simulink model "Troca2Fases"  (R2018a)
settings: Solver=VariableStepAuto  StartTime=0.0  StopTime=200  RelTol=1e-3
undefined symbols (not defined in the file): f7c53156, sdiscope, Troca2Fases

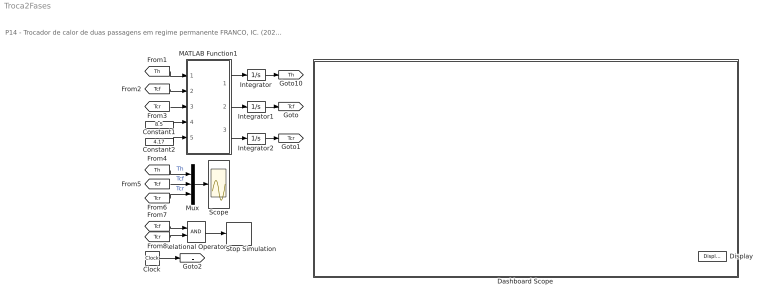
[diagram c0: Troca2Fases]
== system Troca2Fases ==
  note: P14 - Trocador de calor de duas passagens em regime permanente FRANCO, IC. (2022). Modelagem e Simulação: Problemas Típicos da Engenharia Química para Simulação e Análise. NOTAS DE AULA INOVADORAS. The Journal of Engineering and Exact Sciences. Material Complementar.
  Clock : Clock
  Constant1 : Constant  Value=8.5
  Constant2 : Constant  Value=4.17
  Dashboard Scope : Subsystem  DialogController=hmiCreateDDGDialog  IsWebBlock=on  mask(MWDashboardBlock){webBlockId=f7c53156-1038-4bfb-9a74-8fe42874a988, webBlockType=sdiscope, ShowInitialText=on, HMISrcModelName=Troca2Fases}
      mask prompts: webBlockId "WebBlock Id"; webBlockType "WebBlock Type"; HMISrcModelName "Source Model"
      mask help: SimulinkHMI:dialogs:HMIScopeDialogDesc
  Display : DisplayBlock  WebBlockId=332  LabelPosition=Hide  Alignment=Left
  Integrator : Integrator  InitialCondition=80
  Integrator1 : Integrator  InitialCondition=50
  Integrator2 : Integrator  InitialCondition=70
  MATLAB Function1 : MATLAB Function  TreatAsAtomicUnit=on
  Mux : Mux  Inputs=3
  Relational Operator : RelationalOperator  OutDataTypeStr=boolean  RndMeth=Simplest
  Scope : Scope
  Stop Simulation : Stop
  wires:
  MATLAB Function1/1(dTh) -> Integrator/1
  Integrator/1 -> [Th]
  [Th] -> MATLAB Function1/1(Th)
  MATLAB Function1/2(dTcf) -> Integrator1/1
  Integrator1/1 -> [Tcf]
  [Tcf] -> MATLAB Function1/2(Tcf)
  [Tcr] -> MATLAB Function1/3(Tcr)
  MATLAB Function1/3(dTcr) -> Integrator2/1
  Integrator2/1 -> [Tcr]
  Constant1/1 -> MATLAB Function1/4(Wh)
  [Th] -> Mux/1  "Th"
  [Tcf] -> Mux/2  "Tcf"
  Constant2/1 -> MATLAB Function1/5(Wc)
  Mux/1 -> Scope/1
  [Tcr] -> Mux/3  "Tcr"
  Relational Operator/1 -> Stop Simulation/1
  [Tcf] -> Relational Operator/1
  [Tcr] -> Relational Operator/2
  Clock/1 -> [L]

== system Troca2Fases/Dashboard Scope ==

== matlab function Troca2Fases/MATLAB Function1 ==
function [dTh,dTcf,dTcr]=fcn(Th,Tcf,Tcr,Wh,Wc)
%% Parâmetros
Cp  =  4.184;
U   =  1.500;

%% Modelo matemático
dTh = -U*(Th-Tcf)/(2*Wh*Cp)-U*(Th-Tcr)/(2*Wh*Cp);
dTcf=  U*(Th-Tcf)/(2*Wc*Cp);
dTcr= -U*(Th-Tcr)/(2*Wc*Cp);
end
